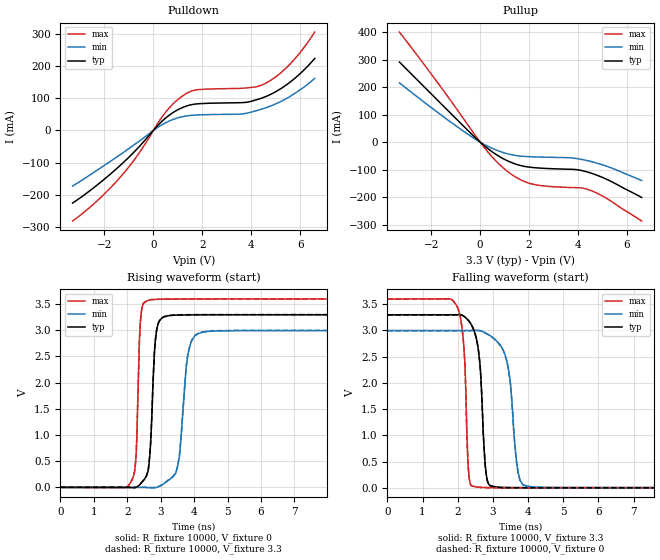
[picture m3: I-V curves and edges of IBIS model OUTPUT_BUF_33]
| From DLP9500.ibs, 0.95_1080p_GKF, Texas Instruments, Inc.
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[Model]   OUTPUT_BUF_33
Model_type  Output
Vref =   0
Rref =   10000
Cref =   0p
Vmeas =   1.5
| variable   typ   min   max
C_comp   3.21pF   1.94pF   4.74pF
| C_pullup   3.64pF   2.66pF   4.74pF
| C_pulldown   2.77pF   1.94pF   3.37pF
[Temperature Range]   40   125   -40
| Ambient temperature   25   110   -40
[Voltage range]   3.3   3   3.6
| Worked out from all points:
|   slope of the pulldown table from 0 to 0.495 V, typ, clamps not added: 13 ohm
|   slope of the pullup table from 0 to 0.495 V, typ, clamps not added: 13.9 ohm
|   rising waveform, R_fixture 10000, V_fixture 0: 20-80 % time 141ps typ, 224ps min, 96.6ps max; typ from 0 V to 3.3 V
|   falling waveform, R_fixture 10000, V_fixture 3.3: 20-80 % time 174ps typ, 253ps min, 128ps max; typ from 3.3 V to 0.004 V
|   rising waveform, R_fixture 10000, V_fixture 3.3: 20-80 % time 141ps typ, 224ps min, 96.6ps max; typ from 0.004 V to 3.3 V
|   falling waveform, R_fixture 10000, V_fixture 0: 20-80 % time 174ps typ, 253ps min, 127ps max; typ from 3.3 V to 0 V
[Pulldown]
| OUTPUT_BUF_33
|   Voltage   I(typ)   I(min)   I(max)
-3.3V     -226.2mA   -173.3mA   -282.1mA
-2.295V   -169.9mA   -123.8mA   -219.2mA
-1.33V    -107.2mA   -74.11mA   -143.8mA
-600mV    -52.22mA   -34.53mA   -72.47mA
410mV     32.56mA    20.25mA    47.77mA
1.075V    67.43mA    40.79mA    100.9mA
1.73V     82.48mA    48.16mA    126.2mA
3.6V      86.84mA    51.43mA    131.6mA
4.555V    104.5mA    69.64mA    145.9mA
5.055V    123.1mA    84.78mA    170.1mA
5.57V     149.4mA    105.4mA    205.6mA
6.6V      224.6mA    162.6mA    306.9mA
[Pullup]
| OUTPUT_BUF_33
|   Voltage   I(typ)   I(min)   I(max)
-3.3V     291.5mA    215.7mA    400.8mA
-1.695V   148.4mA    105.3mA    211.2mA
-290mV    24.16mA    16.15mA    35.77mA
435mV     -31.66mA   -20.35mA   -48.28mA
1.12V     -68.2mA    -42.36mA   -106.7mA
1.64V     -84.88mA   -50.76mA   -136.5mA
2.16V     -92.49mA   -53.53mA   -153.4mA
3.885V    -99.63mA   -59.08mA   -165.8mA
4.2V      -104.5mA   -63.89mA   -167.4mA
4.49V     -111.6mA   -69.7mA    -175mA
5.155V    -134.7mA   -87.26mA   -204mA
6.6V      -201.3mA   -139.9mA   -287.2mA
[Ramp]
| OUTPUT_BUF_33
| variable   typ   min   max
dV/dt_r   1.98/1.49E-10   1.80/2.36E-10   2.16/1.03E-10
dV/dt_f   1.98/1.77E-10   1.80/2.56E-10   2.16/1.29E-10
R_load = 10000
[Rising Waveform]
| OUTPUT_BUF_33
R_fixture =   10000
C_fixture =   0
L_fixture =   0
V_fixture =   0
V_fixture_min = 0
V_fixture_max = 0
|   Time   V(typ)   V(min)   V(max)
0s        920.7pV    4.06nV     601pV
2.14ns    -4.487mV   139.3uV    142.8mV
2.265ns   1.174mV    246.3uV    626.8mV
2.4ns     71.01mV    -37.67uV   3.22V
2.665ns   557.9mV    -4.992mV   3.577V
2.93ns    3.137V     11.71mV    3.591V
3.47ns    3.289V     311.6mV    3.596V
3.815ns   3.293V     2.54V      3.597V
4.225ns   3.295V     2.959V     3.597V
23ns      3.296V     2.994V     3.597V
[Falling Waveform]
| OUTPUT_BUF_33
R_fixture =   10000
C_fixture =   0
L_fixture =   0
V_fixture =   3.3
V_fixture_min = 3
V_fixture_max = 3.6
|   Time   V(typ)   V(min)   V(max)
0s        3.3V       3V         3.6V
1.985ns   3.302V     3V         3.457V
2.18ns    3.271V     3V         2.632V
2.32ns    3.18V      3V         232.1mV
2.5ns     2.923V     3.004V     19.74mV
2.8ns     313.1mV    2.951V     6.608mV
2.98ns    31.35mV    2.876V     4.673mV
3.395ns   6.65mV     2.423V     3.14mV
3.95ns    4.082mV    37.68mV    2.783mV
23ns      3.639mV    5.256mV    2.73mV
[Rising Waveform]
| OUTPUT_BUF_33
R_fixture =   10000
C_fixture =   0
L_fixture =   0
V_fixture =   3.3
V_fixture_min = 3
V_fixture_max = 3.6
|   Time   V(typ)   V(min)   V(max)
0s        3.639mV    5.256mV    2.73mV
2.14ns    -827.2uV   5.394mV    146.2mV
2.265ns   4.91mV     5.498mV    634mV
2.4ns     75.12mV    5.212mV    3.226V
2.665ns   569mV      298.7uV    3.58V
2.93ns    3.143V     17.28mV    3.594V
3.47ns    3.293V     324.1mV    3.599V
3.815ns   3.297V     2.556V     3.6V
4.225ns   3.299V     2.966V     3.6V
23ns      3.3V       3V         3.6V
[Falling Waveform]
| OUTPUT_BUF_33
R_fixture =   10000
C_fixture =   0
L_fixture =   0
V_fixture =   0
V_fixture_min = 0
V_fixture_max = 0
|   Time   V(typ)   V(min)   V(max)
0s        3.296V     2.994V     3.597V
1.985ns   3.298V     2.994V     3.454V
2.18ns    3.267V     2.994V     2.626V
2.32ns    3.176V     2.995V     227.6mV
2.5ns     2.917V     2.998V     16.86mV
2.795ns   335.9mV    2.947V     3.923mV
2.98ns    27.42mV    2.869V     1.925mV
3.395ns   2.962mV    2.413V     406.4uV
3.95ns    435.7uV    31.71mV    52.61uV
23ns      -7.923nV   13.92nV    -5.083nV
